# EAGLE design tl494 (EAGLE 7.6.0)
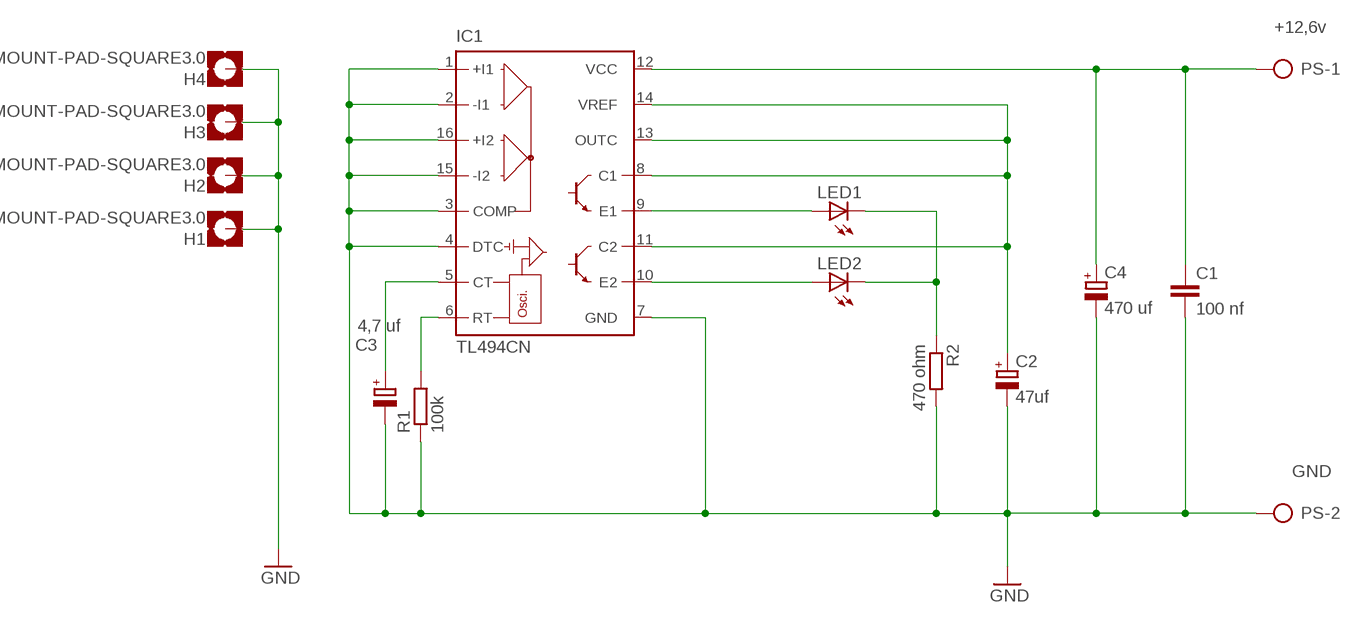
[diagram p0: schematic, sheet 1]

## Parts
C1  100 nf  C-EU050-025X075  [C050-025X075]
C2  47uf  CPOL-EUE2.5-5  [E2,5-5]
C3  4,7 uf  CPOL-EUE2.5-5  [E2,5-5]
C4  470 uf  CPOL-EUE2.5-7  [E2,5-7]
H1  MOUNT-PAD-SQUARE3.0  [3,0-PAD-SQUARE]
H2  MOUNT-PAD-SQUARE3.0  [3,0-PAD-SQUARE]
H3  MOUNT-PAD-SQUARE3.0  [3,0-PAD-SQUARE]
H4  MOUNT-PAD-SQUARE3.0  [3,0-PAD-SQUARE]
IC1  TL494CN  [DIL16]
LED1  LED5MM  [LED5MM]
LED2  LED5MM  [LED5MM]
PS  AK500/2  [AK500/2]
R1  100k  R-EU_0207/10  [0207/10]
R2  470 ohm  R-EU_0207/10  [0207/10]

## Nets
GND: C1.2 C2.- C3.- C4.- H1.B3,0(MOUNT) H2.B3,0(MOUNT) H3.B3,0(MOUNT) H4.B3,0(MOUNT) IC1.1(+I1) IC1.2(-I1) IC1.3(COMP) IC1.4(DTC) IC1.7(GND) IC1.15(-I2) IC1.16(+I2) PS.2 R1.1 R2.2
N$1: LED1.K(C) LED2.K(C) R2.1
N$2: C2.+ IC1.8(C1) IC1.11(C2) IC1.13(OUTC) IC1.14(VREF)
N$3: IC1.9(E1) LED1.A
N$4: IC1.10(E2) LED2.A
N$5: IC1.6(RT) R1.2
N$6: C3.+ IC1.5(CT)
N$10: C1.1 C4.+ IC1.12(VCC) PS.1

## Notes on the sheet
- +12,6v
- GND

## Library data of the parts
C1 = rcl:C-EU: CAPACITOR, European symbol
C2-C4 = rcl:CPOL-EU: POLARIZED CAPACITOR, European symbol
H1-H4 = holes:MOUNT-PAD-SQUARE: MOUNTING PAD, square
IC1 = linear:TL494*: SWITCHMODE Pulse Width Modulation Control Circuit NCV494B http://onsemi.com tl494-d.pdf
LED1 LED2 = led:LED: LED
PS = con-ptr500:AK500/2: CONNECTOR; OC_FARNELL: unknown; OC_NEWARK: unknown
R1 R2 = rcl:R-EU_: RESISTOR, European symbol

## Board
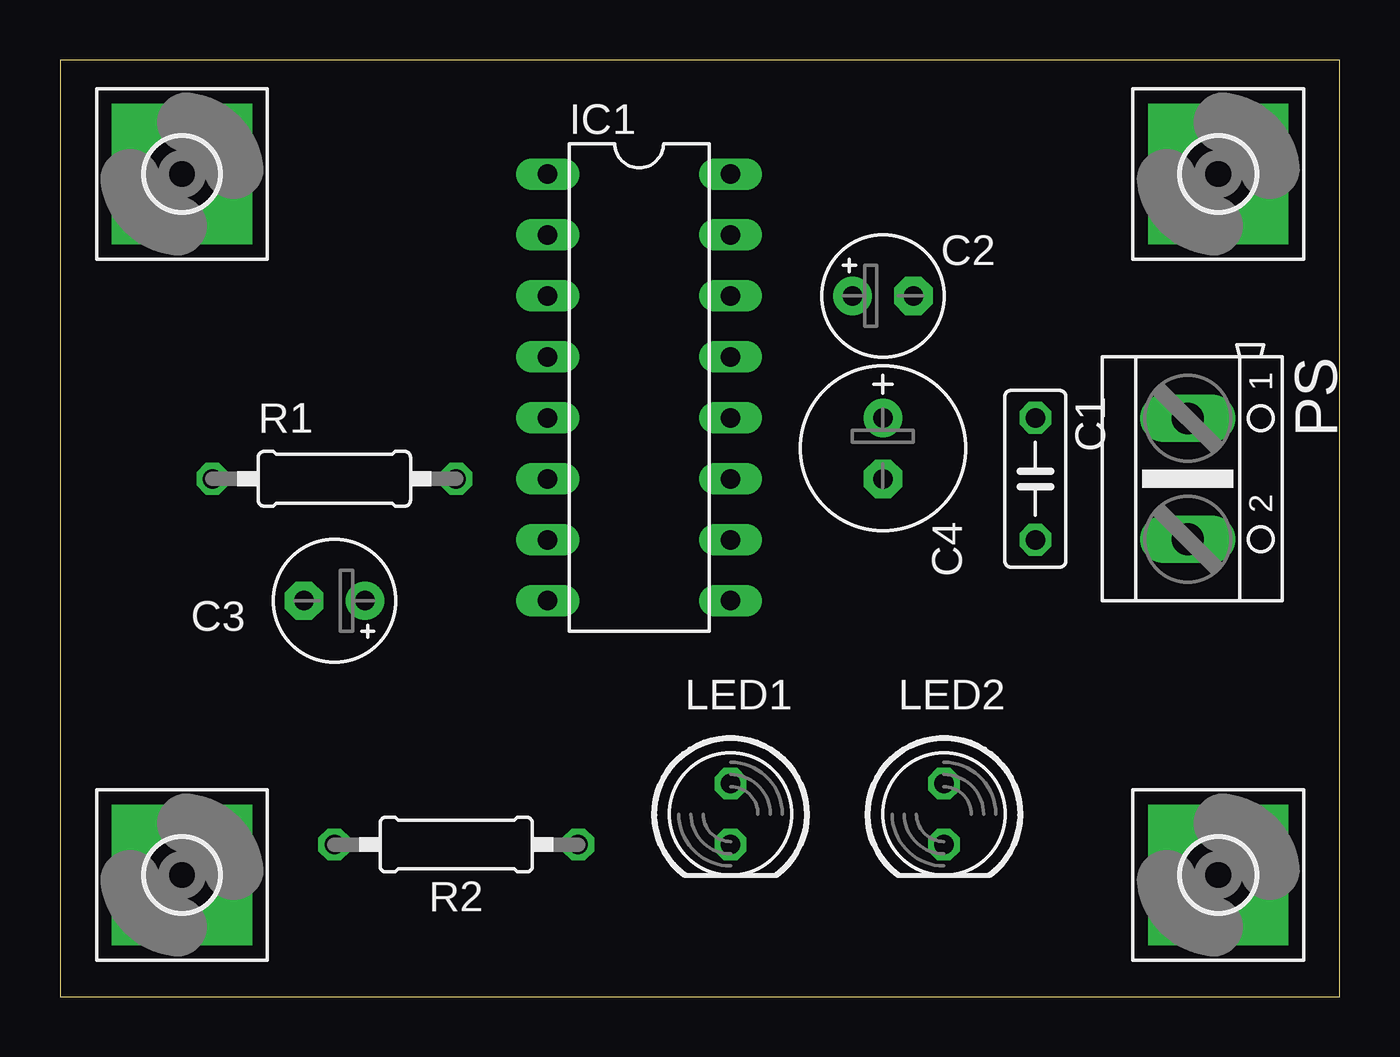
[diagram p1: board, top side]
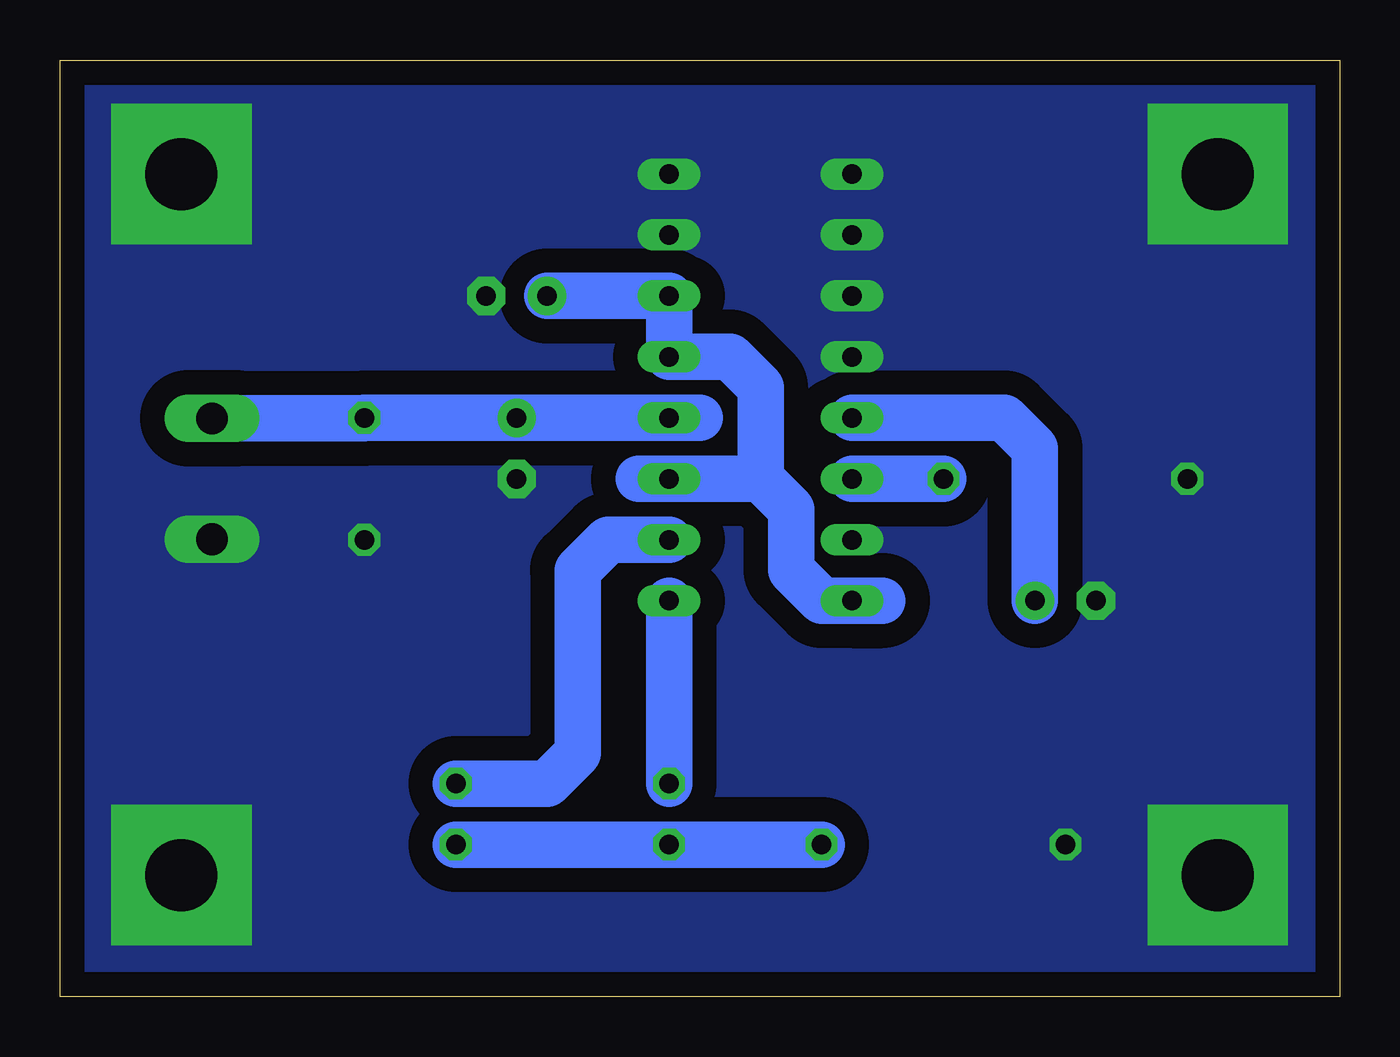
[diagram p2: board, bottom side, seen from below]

Size 53.32 x 39.04 mm. Coordinates in mm from the lower left corner, seen from the top.
Outline: 0,0 53.32,0 53.32,39.04 0,39.04 0,0
Copper layers (1*16): Top 0.035mm / dielectric 1.5mm / Bottom 0.035mm
Design rules "default *": minimum track width 10mil, minimum drill 24mil, track to track 8mil, track to pad 8mil, pad to pad 8mil, via to via 8mil, smd to smd 8mil, copper to edge 40mil, drill to drill 8mil, minimum pad ring 10mil, minimum via ring 8mil, stop-mask expansion 0mil, vias tented up to drill 0mil, thermal gap 0mil

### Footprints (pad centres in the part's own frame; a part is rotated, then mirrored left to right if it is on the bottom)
C050-025X075 = drill 0.813 octagon: 1 -2.54,0; 2 2.54,0
E2,5-5 = drill 0.813 pad 1.6: + -1.27,0 | drill 0.813 pad 1.6 octagon: - 1.27,0
E2,5-7 = drill 0.813 pad 1.6: + -1.27,0 | drill 0.813 pad 1.6 octagon: - 1.27,0
3,0-PAD-SQUARE = drill 3 pad 5.842 square: B3,0 0,0
DIL16 = drill 0.813 long: 1 -8.89,-3.81; 2 -6.35,-3.81; 3 -3.81,-3.81; 4 -1.27,-3.81; 5 1.27,-3.81; 6 3.81,-3.81; 7 6.35,-3.81; 8 8.89,-3.81; 9 8.89,3.81; 10 6.35,3.81; 11 3.81,3.81; 12 1.27,3.81; 13 -1.27,3.81; 14 -3.81,3.81; 15 -6.35,3.81; 16 -8.89,3.81
LED5MM = drill 0.813 octagon: A -1.27,0; K 1.27,0
AK500/2 = drill 1.321 long: 1 -2.515,0; 2 2.515,0
0207/10 = drill 0.813 octagon: 1 -5.08,0; 2 5.08,0

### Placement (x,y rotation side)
C1  40.64,21.59 270 top
C2  34.29,29.21 0 top
C3  11.43,16.51 180 top
C4  34.29,22.86 270 top
H1  48.26,34.29 0 top
H2  48.26,5.08 0 top
H3  5.08,34.29 0 top
H4  5.08,5.08 0 top
IC1  24.13,25.4 270 top
LED1  27.94,7.62 270 top
LED2  36.83,7.62 270 top
PS  46.99,21.59 270 top
R1  11.43,21.59 0 top
R2  16.51,6.35 180 top

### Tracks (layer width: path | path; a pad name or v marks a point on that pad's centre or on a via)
GND
  pour Bottom (isolate 1.016): 0,39.37 53.34,39.37 53.34,0 0,0
N$1
  Bottom 1.93: R2.1 LED1.K LED2.K
N$2
  Bottom 1.93: 19.05,16.51 IC1.8 21.59,16.51 22.86,17.78 22.86,20.32 24.13,21.59 | 24.13,21.59 IC1.11 29.21,21.59 | 24.13,21.59 24.13,25.4 25.4,26.67 IC1.13 IC1.14 C2.+
N$3
  Bottom 1.93: LED1.A IC1.9
N$4
  Bottom 1.93: IC1.10 30.48,19.05 31.75,17.78 31.75,10.16 33.02,8.89 LED2.A
N$5
  Bottom 1.93: IC1.6 R1.2
N$6
  Bottom 1.93: IC1.5 13.97,24.13 12.7,22.86 C3.+
N$10
  Bottom 1.93: PS.1 40.66,24.11 C1.1 C4.+ IC1.12 26.67,24.13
